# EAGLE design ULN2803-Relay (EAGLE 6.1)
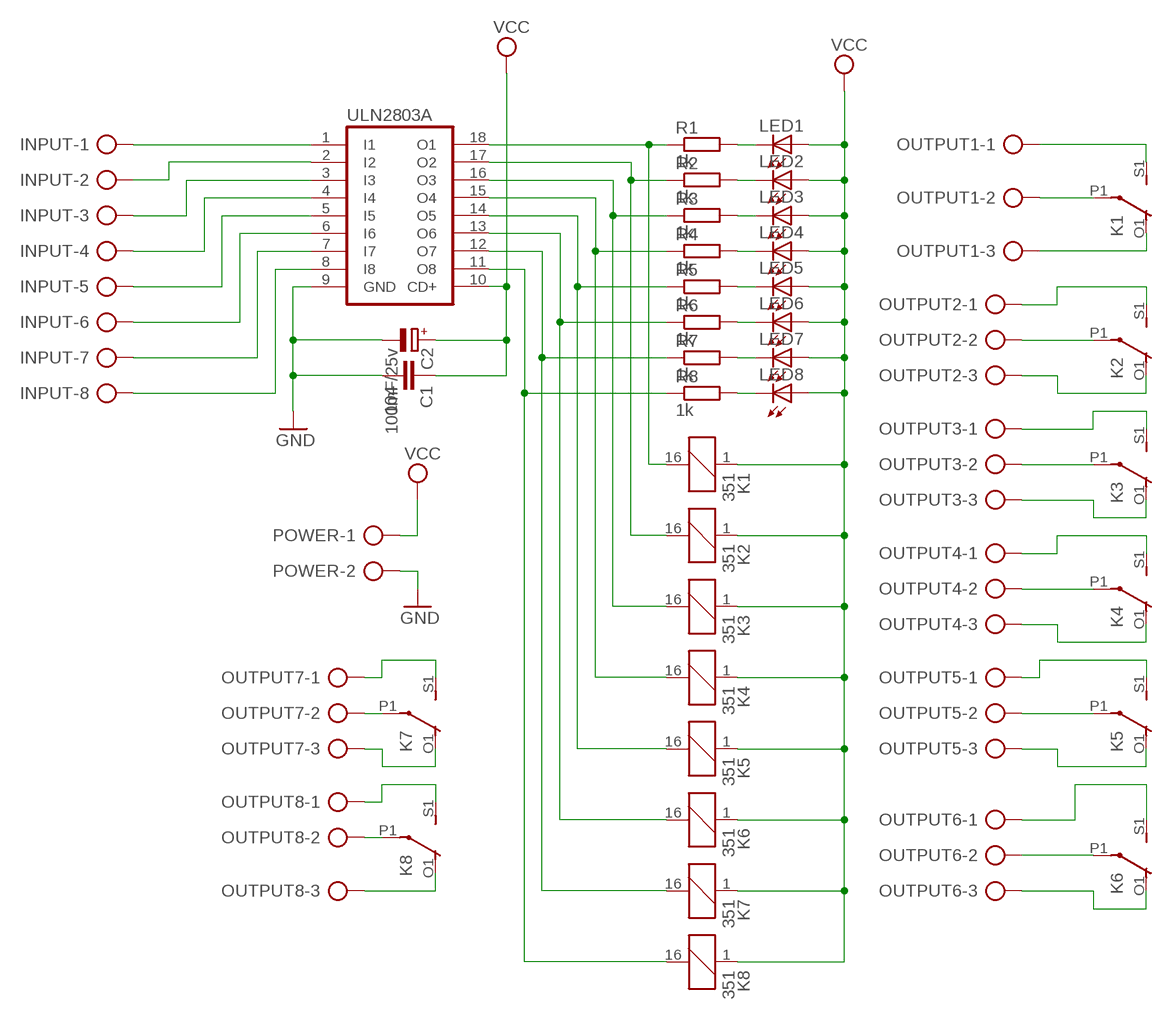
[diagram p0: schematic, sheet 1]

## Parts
C1  104  C2.5/4  [C2.5-4]
C2  100mF/25v  CPOL-EUE2,5-6E  [E2,5-6E]
INPUT  AK500/8  [AK500/8]
K1  351  [351]
K2  351  [351]
K3  351  [351]
K4  351  [351]
K5  351  [351]
K6  351  [351]
K7  351  [351]
K8  351  [351]
LED1  LED5MM  [LED5MM]
LED2  LED5MM  [LED5MM]
LED3  LED5MM  [LED5MM]
LED4  LED5MM  [LED5MM]
LED5  LED5MM  [LED5MM]
LED6  LED5MM  [LED5MM]
LED7  LED5MM  [LED5MM]
LED8  LED5MM  [LED5MM]
OUTPUT1  AK500/3  [AK500/3]
OUTPUT2  AK500/3  [AK500/3]
OUTPUT3  AK500/3  [AK500/3]
OUTPUT4  AK500/3  [AK500/3]
OUTPUT5  AK500/3  [AK500/3]
OUTPUT6  AK500/3  [AK500/3]
OUTPUT7  AK500/3  [AK500/3]
OUTPUT8  AK500/3  [AK500/3]
POWER  AK500/2  [AK500/2]
R1  1k  R-EU_0207/10  [0207/10]
R2  1k  R-EU_0207/10  [0207/10]
R3  1k  R-EU_0207/10  [0207/10]
R4  1k  R-EU_0207/10  [0207/10]
R5  1k  R-EU_0207/10  [0207/10]
R6  1k  R-EU_0207/10  [0207/10]
R7  1k  R-EU_0207/10  [0207/10]
R8  1k  R-EU_0207/10  [0207/10]
ULN2803A  ULN2803A  [DIL18]

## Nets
GND: C1.2 C2.- POWER.2 ULN2803A.9(GND)
N$1: INPUT.1 ULN2803A.1(I1)
N$2: INPUT.2 ULN2803A.2(I2)
N$3: INPUT.3 ULN2803A.3(I3)
N$4: INPUT.4 ULN2803A.4(I4)
N$5: INPUT.5 ULN2803A.5(I5)
N$6: INPUT.6 ULN2803A.6(I6)
N$7: INPUT.7 ULN2803A.7(I7)
N$8: INPUT.8 ULN2803A.8(I8)
N$9: K1.16 R1.1 ULN2803A.18(O1)
N$10: K2.16 R2.1 ULN2803A.17(O2)
N$11: K3.16 R3.1 ULN2803A.16(O3)
N$12: K4.16 R4.1 ULN2803A.15(O4)
N$13: K5.16 R5.1 ULN2803A.14(O5)
N$14: K6.16 R6.1 ULN2803A.13(O6)
N$15: K7.16 R7.1 ULN2803A.12(O7)
N$16: K8.16 R8.1 ULN2803A.11(O8)
N$17: LED1.K(C) R1.2
N$18: LED2.K(C) R2.2
N$19: LED3.K(C) R3.2
N$20: LED4.K(C) R4.2
N$21: LED5.K(C) R5.2
N$22: LED6.K(C) R6.2
N$23: LED7.K(C) R7.2
N$24: LED8.K(C) R8.2
N$25 [OUTPUT]: K1.P1(2:P) OUTPUT1.2
N$26 [OUTPUT]: K1.S1(2:S) OUTPUT1.1
N$27 [OUTPUT]: K1.O1(2:O) OUTPUT1.3
N$28 [OUTPUT]: K2.P1(2:P) OUTPUT2.2
N$29: K2.S1(2:S) OUTPUT2.1
N$30: K2.O1(2:O) OUTPUT2.3
N$31: K7.P1(2:P) OUTPUT7.2
N$32: K7.S1(2:S) OUTPUT7.1
N$33: K7.O1(2:O) OUTPUT7.3
N$34: K8.S1(2:S) OUTPUT8.1
N$35: K8.P1(2:P) OUTPUT8.2
N$36: K8.O1(2:O) OUTPUT8.3
N$37: K3.P1(2:P) OUTPUT3.2
N$38: K3.S1(2:S) OUTPUT3.1
N$39: K3.O1(2:O) OUTPUT3.3
N$40: K4.S1(2:S) OUTPUT4.1
N$41: K4.P1(2:P) OUTPUT4.2
N$42 [OUTPUT]: K4.O1(2:O) OUTPUT4.3
N$43: K5.P1(2:P) OUTPUT5.2
N$44: K5.S1(2:S) OUTPUT5.1
N$45: K5.O1(2:O) OUTPUT5.3
N$46: K6.S1(2:S) OUTPUT6.1
N$47: K6.P1(2:P) OUTPUT6.2
N$48: K6.O1(2:O) OUTPUT6.3
VCC: C1.1 C2.+ K1.1 K2.1 K3.1 K4.1 K5.1 K6.1 K7.1 K8.1 LED1.A LED2.A LED3.A LED4.A LED5.A LED6.A LED7.A LED8.A POWER.1 ULN2803A.10(CD+)
Unconnected: K1.O2(3:O) K1.P2(3:P) K1.S2(3:S) K2.O2(3:O) K2.P2(3:P) K2.S2(3:S) K3.O2(3:O) K3.P2(3:P) K3.S2(3:S) K4.O2(3:O) K4.P2(3:P) K4.S2(3:S) K5.O2(3:O) K5.P2(3:P) K5.S2(3:S) K6.O2(3:O) K6.P2(3:P) K6.S2(3:S) K7.O2(3:O) K7.P2(3:P) K7.S2(3:S) K8.O2(3:O) K8.P2(3:P) K8.S2(3:S)

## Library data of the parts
C1 = capacitor-wima:C: CAPACITOR
C2 = rcl:CPOL-EU: POLARIZED CAPACITOR, European symbol
INPUT = con-ptr500:AK500/8: CONNECTOR; OC_FARNELL: unknown; OC_NEWARK: unknown
K1-K8 = relay:351: RELAY 2 x switch, Omron; OC_FARNELL: unknown; OC_NEWARK: unknown
LED1-LED8 = led:LED: LED
OUTPUT1-OUTPUT8 = con-ptr500:AK500/3: CONNECTOR; OC_FARNELL: unknown; OC_NEWARK: unknown
POWER = con-ptr500:AK500/2: CONNECTOR; OC_FARNELL: unknown; OC_NEWARK: unknown
R1-R8 = resistor:R-EU_: RESISTOR, European symbol
ULN2803A = uln-udn:ULN2803A: DRIVER ARRAY

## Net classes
0 GND: width 0.635 mm
1 OUTPUT: width 0.762 mm

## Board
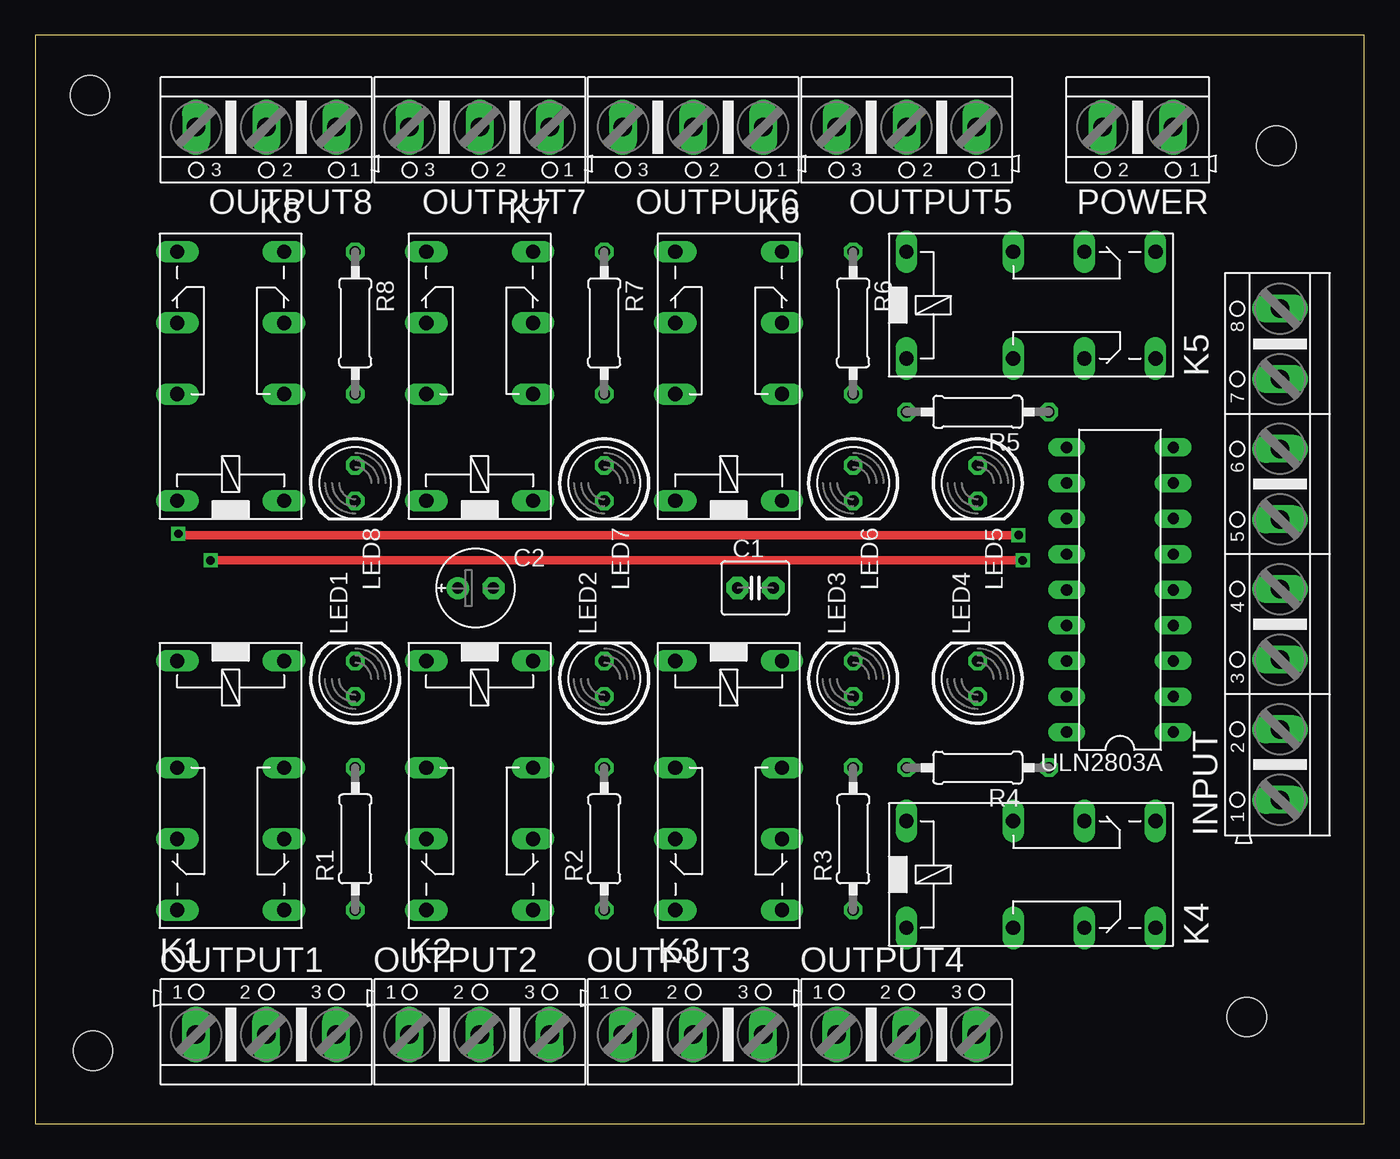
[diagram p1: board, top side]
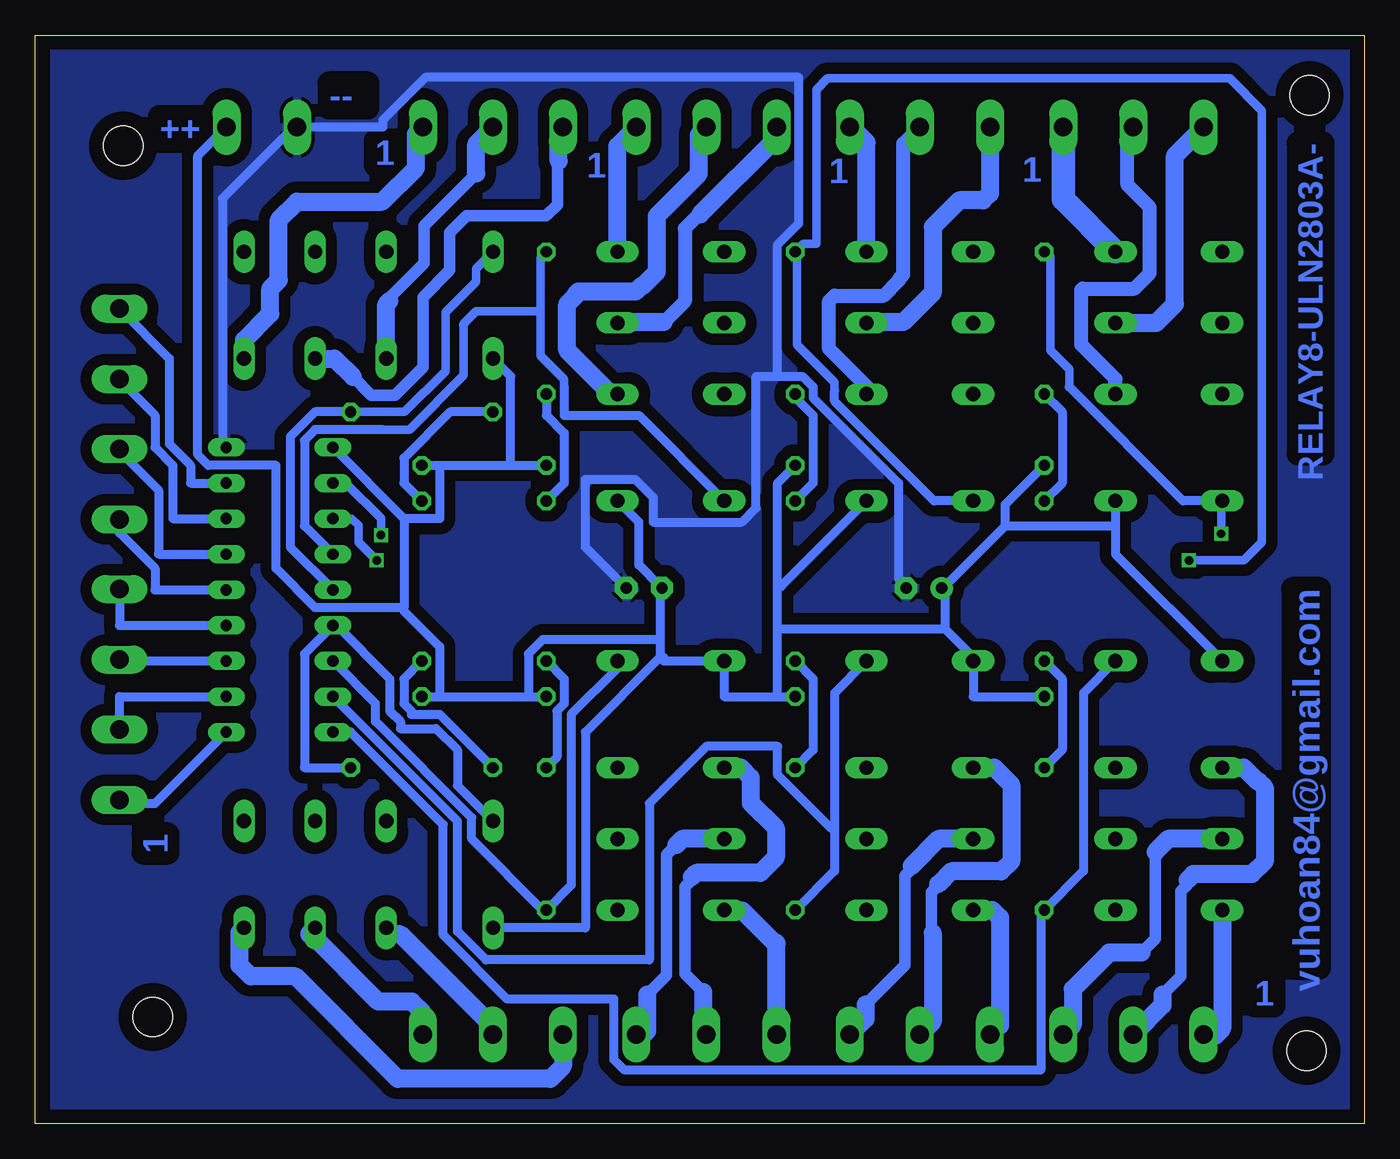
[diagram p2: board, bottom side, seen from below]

Size 94.93 x 77.7 mm. Coordinates in mm from the lower left corner, seen from the top.
Outline: 0,0 94.93,0 94.93,77.7 0,77.7 0,0
Copper layers (1*16): Top 0.035mm / dielectric 1.5mm / Bottom 0.035mm
Design rules: minimum track width 10mil, minimum drill 24mil, track to track 8mil, track to pad 8mil, pad to pad 8mil, via to via 8mil, smd to smd 8mil, copper to edge 40mil, drill to drill 8mil, minimum pad ring 10mil, minimum via ring 8mil, stop-mask expansion 4mil, vias tented up to drill 0mil, thermal gap 10mil
Holes 2.8 mm at 4.13,5.2 86.53,7.6 88.63,69.8 3.93,73.4

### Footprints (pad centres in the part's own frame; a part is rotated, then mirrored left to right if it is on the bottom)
C2.5-4 = drill 0.813 pad 1.6 octagon: 1 -1.27,0; 2 1.27,0
E2,5-6E = drill 0.813 pad 1.575: + -1.27,0 | drill 0.813 pad 1.575 octagon: - 1.27,0
AK500/8 = drill 1.321 long: 1 -17.526,0; 2 -12.497,0; 3 -7.518,0; 4 -2.489,0; 5 2.489,0; 6 7.518,0; 7 12.497,0; 8 17.526,0
351 = drill 1.016 long: 1 -3.81,-3.81; 16 -3.81,3.81; O1 8.89,-3.81; O2 8.89,3.81; P1 3.81,-3.81; P2 3.81,3.81; S1 13.97,-3.81; S2 13.97,3.81
LED5MM = drill 0.813 octagon: A -1.27,0; K 1.27,0
AK500/3 = drill 1.321 long: 1 -5.004,0; 2 0,0; 3 5.004,0
AK500/2 = drill 1.321 long: 1 -2.515,0; 2 2.515,0
0207/10 = drill 0.813 octagon: 1 -5.08,0; 2 5.08,0
DIL18 = drill 0.813 long: 1 -10.16,-3.81; 2 -7.62,-3.81; 3 -5.08,-3.81; 4 -2.54,-3.81; 5 0,-3.81; 6 2.54,-3.81; 7 5.08,-3.81; 8 7.62,-3.81; 9 10.16,-3.81; 10 10.16,3.81; 11 7.62,3.81; 12 5.08,3.81; 13 2.54,3.81; 14 0,3.81; 15 -2.54,3.81; 16 -5.08,3.81; 17 -7.62,3.81; 18 -10.16,3.81

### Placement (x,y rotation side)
C1  51.43,38.24 0 top
C2  31.46,38.22 0 top
INPUT  88.9,40.64 90 top
K1  13.97,29.21 270 top
K2  31.75,29.21 270 top
K3  49.53,29.21 270 top
K4  66.04,17.78 0 top
K5  66.04,58.42 0 top
K6  49.53,48.26 90 top
K7  31.75,48.26 90 top
K8  13.97,48.26 90 top
LED1  22.86,31.75 90 top
LED2  40.64,31.75 90 top
LED3  58.42,31.75 90 top
LED4  67.31,31.75 90 top
LED5  67.31,45.72 270 top
LED6  58.42,45.72 270 top
LED7  40.64,45.72 270 top
LED8  22.86,45.72 270 top
OUTPUT1  16.51,6.35 0 top
OUTPUT2  31.75,6.35 0 top
OUTPUT3  46.99,6.35 0 top
OUTPUT4  62.23,6.35 0 top
OUTPUT5  62.23,71.12 180 top
OUTPUT6  46.99,71.12 180 top
OUTPUT7  31.75,71.12 180 top
OUTPUT8  16.51,71.12 180 top
POWER  78.74,71.12 180 top
R1  22.86,20.32 90 top
R2  40.64,20.32 90 top
R3  58.42,20.32 90 top
R4  67.31,25.4 180 top
R5  67.31,50.8 180 top
R6  58.42,57.15 270 top
R7  40.64,57.15 270 top
R8  22.86,57.15 270 top
ULN2803A  77.47,38.1 90 top

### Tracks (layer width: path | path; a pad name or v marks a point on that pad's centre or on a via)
GND
  Bottom 0.635: ULN2803A.9 81.53,48.51 81.53,66.04 76.45,71.12 POWER.2 70.1,71.12 70.1,71.63 67.06,74.68 40.39,74.68 40.39,64.26 41.91,62.74 41.91,53.34 | 41.91,53.34 43.43,53.34 43.43,43.94 44.45,42.93 50.8,42.93 50.8,44.7 52.07,45.97 55.63,45.97 55.63,41.15 52.83,38.35 C1.2 | 41.91,53.34 40.13,53.34 39.37,52.58 39.37,51.82 33.27,45.72 33.27,38.86 32.77,38.35 C2.-
  pour Bottom (isolate 0.813, rank 6): 1.13,77.1 93.83,77.1 93.83,1.1 0.93,1.1 0.93,76.9
N$1
  Bottom 0.635: ULN2803A.1 86.36,22.86 88.9,22.86 INPUT.1
N$2
  Bottom 0.635: ULN2803A.2 88.9,30.48 INPUT.2
N$3
  Bottom 0.635: ULN2803A.3 88.9,33.02 INPUT.3
N$4
  Bottom 0.635: ULN2803A.4 88.9,35.56 INPUT.4
N$5
  Bottom 0.635: ULN2803A.5 86.36,38.1 86.36,39.62 88.9,42.16 INPUT.5
N$6
  Bottom 0.635: ULN2803A.6 86.11,40.64 86.11,45.21 88.9,48.01 INPUT.6
N$7
  Bottom 0.635: ULN2803A.7 85.09,43.18 85.09,46.99 86.36,48.26 86.36,50.55 88.9,53.09 INPUT.7
N$8
  Bottom 0.635: ULN2803A.8 83.82,45.72 83.82,46.99 85.34,48.51 85.34,54.61 INPUT.8
N$9
  Bottom 0.635: K1.16 20.07,30.73 20.07,18.03 R1.1 23.11,15.24 23.11,3.81 52.83,3.81 53.59,4.57 53.59,8.89 61.21,8.89 65.79,13.46 65.79,21.34 72.39,27.94 ULN2803A.18
N$10
  Bottom 0.635: R2.1 37.85,18.03 37.85,21.08 | 37.85,21.08 37.85,30.73 K2.16 | ULN2803A.17 64.77,21.59 64.77,13.72 62.74,11.68 51.05,11.68 51.05,22.86 46.99,26.92 41.91,26.92 41.91,24.89 38.1,21.08 37.85,21.08
N$11
  Bottom 0.635: K3.16 53.34,32.51 56.64,29.21 56.64,17.02 R3.1 58.67,15.24 63.75,20.32 63.75,21.84 70.61,28.7 70.61,29.97 ULN2803A.16
N$12
  Bottom 0.635: R4.1 75.69,25.4 75.69,33.53 ULN2803A.15 73.41,35.56 69.6,31.75 69.6,29.46 68.83,28.7 68.83,28.19 66.29,28.19 64.77,26.67 64.77,24.13 K4.16
N$13
  Bottom 0.61: R5.1 68.53,50.8 65.63,53.7 65.63,57.9 63.43,60.1 63.43,61.03 K5.16
  Bottom 0.635: ULN2803A.14 76.71,41.15 76.71,49.02 74.93,50.8 R5.1
N$14
  Bottom 0.61: 70.12,49.53 68.2,49.53 64.33,53.4 64.33,57 | 57.15,52.58 57.15,53.12 58.83,54.8 58.83,57.9 | 58.83,57.9 58.83,61.8 R6.1 58.33,62.3 | 64.33,57.1 64.27,57.16 63.43,58 58.93,58 58.83,57.9
  Bottom 0.635: ULN2803A.13 75.69,42.67 75.69,48.77 74.93,49.53 70.12,49.53 | K6.16 51.82,50.55 57.15,50.55 57.15,52.58 | R6.1 | 64.27,57.16 64.26,57.15 64.33,57
N$15  (via drill 0.6)
  Top 0.61: v70.53,40.2 v12.53,40.2
  Bottom 0.61: ULN2803A.12 72.31,43.18 71.83,42.7 71.83,41.5 v70.53,40.2 | v12.53,40.2 8.63,40.2 7.33,41.5 7.33,72.3 9.63,74.6 38.33,74.6 39.13,73.8 39.13,62.8 40.07,62.8 R7.1 | 37.85,52.32 37.85,52.92 40.53,55.6 40.53,61.98 40.53,62.2 40.73,62.4
  Bottom 0.635: 37.85,52.32 37.85,51.56 30.73,44.45 K7.16 | 40.53,61.98 40.64,61.98 R7.1
N$16  (via drill 0.6)
  Top 0.61: v70.23,42 10.33,42 v10.23,42.1
  Bottom 0.61: ULN2803A.11 72.75,45.72 70.23,43.2 v70.23,42 | v10.23,42.1 10.23,44.38 K8.16 | 21.08,52.58 21.08,53.85 22.43,55.2 22.43,61.9 22.73,62.2
  Bottom 0.635: 21.08,52.58 12.95,44.45 K8.16 | R8.1 22.73,62.2
N$17
  Bottom 0.635: R1.2 21.59,26.67 21.59,31.75 LED1.K
N$18
  Bottom 0.635: R2.2 39.37,26.67 39.37,31.75 LED2.K
N$19
  Bottom 0.635: R3.2 57.66,26.16 57.66,29.46 57.15,29.97 57.15,31.75 LED3.K
N$20
  Bottom 0.635: R4.2 66.04,29.21 68.07,29.21 68.07,29.46 68.58,29.97 68.58,31.75 LED4.K
N$21
  Bottom 0.635: LED5.K 68.58,45.72 68.58,47.5 65.28,50.8 R5.2
N$22
  Bottom 0.635: LED6.K 57.15,45.72 57.15,49.28 58.42,50.55 R6.2
N$23
  Bottom 0.635: LED7.K 39.37,45.72 39.37,50.55 40.64,51.82 R7.2
N$24
  Bottom 0.635: LED8.K 21.59,45.72 21.59,50.8 R8.2
N$25
  Bottom 0.813: 12.63,17.4 12.63,17.1 13.13,16.6 13.13,10.5 14.43,9.2
  Bottom 1.27: K1.P1 8.63,25.4 7.63,24.4 7.53,24.4 7.13,24 7.13,18.7 8.03,17.8 12.23,17.8 12.63,17.4 | 14.43,9.2 14.43,8.43 OUTPUT1.2
N$26
  Bottom 0.762: OUTPUT1.1 11.68,6.35 11.33,6.2
  Bottom 1.27: K1.S1 10.16,6.77 10.73,6.2 11.33,6.2
N$27
  Bottom 0.813: 14.93,19.4 14.93,13.2 15.93,12.2
  Bottom 1.27: K1.O1 14.01,20.32 14.93,19.4 | 15.93,12.2 18.23,12.2 20.83,9.6 20.83,7.03 OUTPUT1.3
N$28
  Bottom 0.813: 30.43,17.1 30.43,17 30.93,16.5 30.93,13.7 30.83,13.6
  Bottom 1.27: K2.P1 26.43,25.4 25.23,24.2 25.23,18.7 25.93,18 29.53,18 30.43,17.1 | 30.83,13.6 30.83,7.27 OUTPUT2.2
N$29
  Bottom 0.635: OUTPUT2.1 26.92,6.35 26.63,6.4
  Bottom 1.27: K2.S1 26.57,15.24 26.03,14.7 26.03,7 26.63,6.4
N$30
  Bottom 0.813: 32.33,18.4 32.33,18.2 32.83,17.7 32.83,11.3 35.63,8.5
  Bottom 1.27: K2.O1 30.41,20.32 32.33,18.4 | 35.63,8.5 35.63,7.47 OUTPUT2.3
N$31
  Bottom 1.016: K7.P1 35.56,52.63 38.23,55.3 38.23,58.7 37.83,59.1 34.33,59.1 33.23,60.2 33.23,60.3 32.93,60.6 32.93,69.94 OUTPUT7.2
N$32
  Bottom 0.635: OUTPUT7.1 36.83,71.12 36.74,71.21
  Bottom 1.27: K7.S1 35.56,70.03 36.74,71.21 36.83,71.3
N$33
  Bottom 1.27: OUTPUT7.3 26.75,66.38 27.23,65.9 28.93,65.9 30.83,64 30.83,59.3 32.93,57.2 35.51,57.2 K7.O1
N$34
  Bottom 1.676: OUTPUT8.1 21.51,65.96 K8.S1
N$35
  Bottom 1.016: K8.P1 17.78,53.15 20.23,55.6 20.23,59.5 20.13,59.6 16.43,59.6 15.33,60.7 15.33,65.4 16.93,67 16.93,70.7 OUTPUT8.2
N$36
  Bottom 1.27: K8.O1 14.88,57.15 13.53,58.5 13.53,69.1 OUTPUT8.3
N$37
  Bottom 0.813: 48.03,17.6 48.03,17.4 48.53,16.9 48.53,10.7 47.23,9.4
  Bottom 1.27: K3.P1 44.53,25.4 43.83,24.7 43.83,22.9 42.03,21.1 42.03,19 43.13,17.9 47.73,17.9 48.03,17.6 | 47.23,9.4 47.23,6.59 OUTPUT3.2
N$38
  Bottom 0.635: K3.S1 45.72,15.2
  Bottom 1.27: OUTPUT3.1 41.99,12.86 42.13,13 42.23,13 44.43,15.2 45.72,15.2 45.93,15.2
N$39
  Bottom 0.635: OUTPUT3.3 52.07,6.35 51.73,6.1
  Bottom 0.813: 49.13,19.9 49.83,19.2 49.83,10.6 51.23,9.2
  Bottom 1.27: K3.O1 48.71,20.32 49.13,19.9 | 51.23,9.2 51.23,6.6 51.73,6.1
N$40
  Bottom 1.27: OUTPUT4.1 57.23,4.1 58.13,3.2 69.03,3.2 76.33,10.5 79.53,10.5 80.33,11.3 80.33,13.65 K4.S1
N$41
  Bottom 1.27: OUTPUT4.2 62.23,6.9 68.83,13.5 69.38,13.5 K4.P1
N$42
  Bottom 1.27: OUTPUT4.3 67.23,7.9 68.03,8.7 70.43,8.7 75.23,13.5 75.33,13.5 75.33,13.57 K4.O1
N$43
  Bottom 0.813: 69.63,58.7 69.63,58.9 67.13,61.4 67.13,64.1 63.43,67.8
  Bottom 1.27: K5.P1 69.85,58.48 69.63,58.7 | 63.43,67.8 63.43,69.92 OUTPUT5.2
N$44
  Bottom 1.27: K5.S1 80.01,55.92 78.13,57.8 78.13,59.6 77.53,60.2 77.53,64.5 76.23,65.8 70.13,65.8 67.73,68.2 67.73,70.62 OUTPUT5.1
N$45
  Bottom 0.813: 72.23,53.3 70.93,52 69.23,52 67.23,54 67.23,59 65.33,60.9 65.33,63.6 64.13,64.8 58.43,64.8 57.63,65.6 57.63,68.6 57.53,68.7
  Bottom 1.27: K5.O1 73.54,54.61 72.23,53.3 | 57.53,68.7 57.53,70.82 OUTPUT5.3
N$46
  Bottom 1.27: K6.S1 53.34,69.77 OUTPUT6.1
N$47
  Bottom 1.27: K6.P1 53.8,52.07 56.93,55.2 56.93,58.5 56.33,59.1 56.33,59.2 56.13,59.4 52.03,59.4 51.63,59.8 51.53,59.8 50.53,60.8 50.53,64.8 47.53,67.8 47.53,70.58 OUTPUT6.2
N$48
  Bottom 1.016: 47.43,64.9 47.53,64.9 48.53,63.9 48.53,58.7 50.03,57.2
  Bottom 1.27: OUTPUT6.3 41.99,70.34 47.43,64.9 | 50.03,57.2 53.29,57.2 K6.O1
VCC
  Bottom 0.635: LED4.A 66.04,30.48 | 66.04,30.48 59.69,30.48 | 59.69,30.48 LED3.A | LED5.A 66.04,46.99 | 66.04,46.99 60.96,46.99 | 60.96,46.99 LED6.A | 68.58,43.18 ULN2803A.10 | 68.58,43.18 66.04,43.18 66.04,46.99 | K5.1 60.96,53.34 60.96,46.99 | 68.58,36.83 74.93,36.83 77.72,39.62 77.72,46.99 82.55,46.99 83.31,47.75 83.31,69.09 81.28,71.12 POWER.1 | 68.58,43.18 68.58,36.83 | 66.04,30.48 66.04,34.04 68.58,36.58 68.58,36.83 | K1.1 17.78,40.64 17.78,42.67 | K8.1 17.78,42.67 | LED1.A 27.94,30.48 K2.1 27.94,33.27 29.97,35.31 | LED8.A 25.65,44.2 25.65,42.67 | 25.65,42.67 29.97,38.35 C2.+ 29.97,38.1 29.97,35.31 | 25.65,42.67 17.78,42.67 | 41.91,30.48 45.72,30.48 K3.1 50.04,33.02 50.04,33.27 50.29,33.27 | 41.91,30.48 LED2.A | LED7.A 41.91,45.72 41.91,38.35 | 41.91,30.48 41.91,35.31 | 41.91,35.31 41.91,38.35 | K7.1 41.66,38.35 41.91,38.35 | K4.1 55.63,13.97 55.63,27.94 50.29,33.27 | 50.29,34.54 50.29,38.1 C1.1 50.29,38.35 51.82,39.88 51.82,42.93 K6.1 | 50.29,34.54 50.29,33.27 | 41.91,35.31 29.97,35.31 | 59.69,30.48 59.69,33.53 58.67,34.54 50.29,34.54

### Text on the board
Bottom: -- | RELAY8-ULN2803A- | ++ | 1 | 1 | 1 | 1 | vuhoan84@gmail.com | 1 | 1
